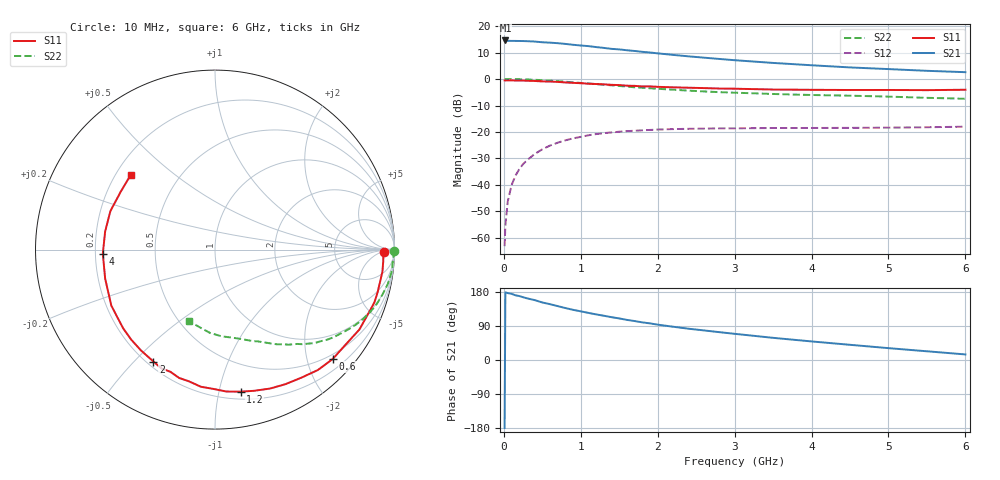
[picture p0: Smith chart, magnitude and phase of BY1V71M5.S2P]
! SIEMENS Small Signal Semiconductors
! BFY420
! Si NPN RF SIEGET Grounded Emitter Transistor in MICRO-X
! VCE = 1.75 V  IC = 1.5 mA
! Common Emitter S-Parameters:  October  1996
# GHz  S  MA  R  50
!  f  S11  S21  S12  S22
! GHz  MAG  ANG  MAG  ANG  MAG  ANG  MAG  ANG
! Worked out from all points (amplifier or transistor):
!   36 points, 10 MHz to 6 GHz, reference 50 ohm
!   highest |S21| = 14.6 dB at 20 MHz (marker M1)
!   |S21| within 3 dB of that: start of sweep to 1.352 GHz
!   unconditionally stable (mu >= 1): 4.257 GHz to end of sweep
!   at 250 MHz: K = 0.05, MSG = 23.2 dB, |S12| = -32.1 dB
!   at 1.4 GHz: K = 0.25, MSG = 15.8 dB, |S12| = -20.2 dB
!   at 6 GHz: K = 1.29, MAG = 7.1 dB, |S12| = -18.0 dB
!   S11 on the Smith chart (normalised r, x): 10 MHz: 32, -8; 600 MHz: 0.40, -2.49; 1.2 GHz: 0.26, -1.16; 2 GHz: 0.23, -0.57; 4 GHz: 0.23, -0.02; 6 GHz: 0.26, +0.36
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0.01  0.9429 -0.9  5.332 -179.4  0.0007 94.3  0.9971 -0.4
0.02  0.9383 -1.6  5.342 178.6  0.0017 94.8  0.9927 -0.7
0.05  0.9396 -3.8  5.257 176.6  0.0048 83.2  0.9956 -1.8
0.1  0.9409 -7.5  5.24 174.7  0.0099 89.1  0.9923 -3.7
0.15  0.9371 -10.9  5.234 170.8  0.0149 82.7  0.993 -5.7
0.2  0.9367 -14.8  5.221 168.8  0.0198 81.8  0.9909 -7.5
0.25  0.9352 -18.4  5.207 165.7  0.0248 78.5  0.9854 -9.4
0.4  0.9194 -29.0  5.094 158.1  0.0384 72.7  0.9666 -14.9
0.5  0.9 -36.0  4.941 151.8  0.0471 68.2  0.9513 -18.4
0.6  0.8955 -42.9  4.854 147.3  0.0554 64.8  0.9329 -21.8
0.8  0.8607 -56.0  4.597 137.1  0.0697 56.5  0.889 -28.1
1.1  0.8163 -74.5  4.176 124.3  0.0867 47.0  0.8225 -36.3
1.2  0.8042 -79.8  4.006 120.3  0.0913 44.1  0.8014 -38.8
1.6  0.7483 -101.1  3.489 105.8  0.1038 34.0  0.7185 -47.2
2  0.7118 -118.8  3.051 93.3  0.1112 26.4  0.6534 -53.8
2.2  0.6969 -126.3  2.853 87.8  0.1134 23.1  0.6296 -56.9
2.8  0.6612 -145.8  2.392 73.5  0.1171 16.0  0.5648 -64.9
3.5  0.633 -165.2  2.012 58.5  0.1189 10.6  0.5218 -73.1
4  0.6255 -177.9  1.818 49.0  0.1192 7.9  0.4993 -79.1
4.5  0.6203 170.7  1.655 40.1  0.1197 5.9  0.4847 -85.6
5.5  0.6163 148.6  1.428 23.0  0.1229 4.2  0.4415 -101.0
6  0.6275 138.5  1.346 14.7  0.1261 3.9  0.4238 -109.8
